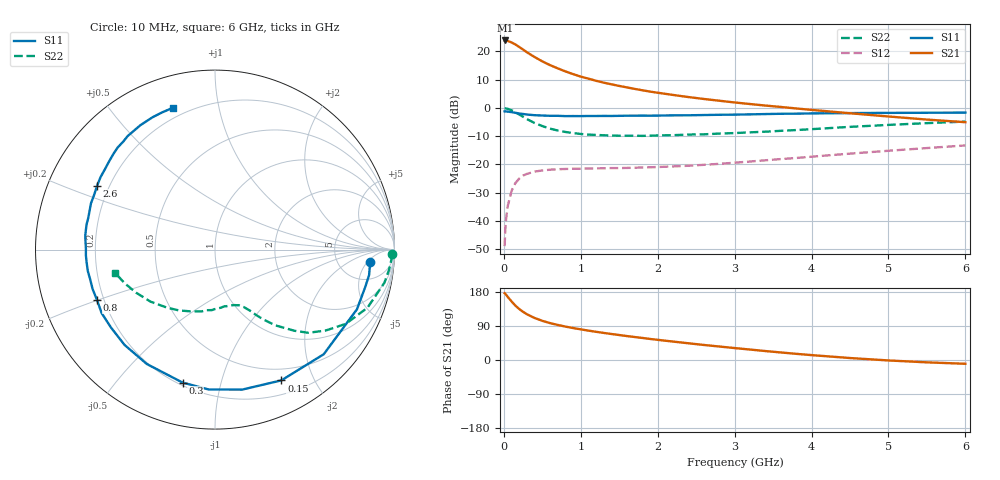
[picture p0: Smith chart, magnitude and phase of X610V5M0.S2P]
! SIEMENS Small Signal Semiconductors
! BFP193W
! Si NPN RF Bipolar Junction Transistor in SOT343
! VCE = 10 V  IC = 5 mA
! Common Emitter S-Parameters:  April 1994
# GHz  S  MA  R  50
!  f  S11  S21  S12  S22
! GHz  MAG  ANG  MAG  ANG  MAG  ANG  MAG  ANG
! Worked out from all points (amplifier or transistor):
!   40 points, 10 MHz to 6 GHz, reference 50 ohm
!   highest |S21| = 23.8 dB at 20 MHz (marker M1)
!   |S21| within 3 dB of that: start of sweep to 237.7 MHz
!   unconditionally stable (mu >= 1): 1.756 GHz to 4.541 GHz
!   at 200 MHz: K = 0.14, MSG = 23.2 dB, |S12| = -25.0 dB
!   at 1.5 GHz: K = 0.90, MSG = 14.5 dB, |S12| = -21.3 dB
!   at 6 GHz: K = 0.92, MSG = 4.1 dB, |S12| = -13.3 dB
!   S11 on the Smith chart (normalised r, x): 10 MHz: 11, -6; 150 MHz: 0.36, -1.57; 300 MHz: 0.22, -0.76; 800 MHz: 0.17, -0.20; 2.6 GHz: 0.15, +0.25; 6 GHz: 0.15, +0.74
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0.01  0.8672 -4.5  15.48 176.3  0.0036 85.0  0.9883 -1.5
0.02  0.8702 -9.3  15.52 174.5  0.0074 83.6  0.9813 -4.7
0.05  0.858 -22.8  15.22 166.8  0.0182 77.0  0.9617 -11.1
0.1  0.8408 -43.9  14.33 154.6  0.034 66.7  0.9089 -20.9
0.15  0.8171 -63.1  13.19 143.5  0.0469 57.8  0.8376 -29.6
0.2  0.7946 -79.0  11.89 134.5  0.0563 50.8  0.7635 -36.2
0.25  0.78 -92.6  10.71 127.1  0.0636 44.8  0.6967 -41.7
0.3  0.7626 -103.7  9.602 120.7  0.0682 39.9  0.633 -45.6
0.4  0.742 -120.8  7.902 110.9  0.0748 33.2  0.5403 -51.4
0.5  0.7322 -133.5  6.64 103.4  0.0784 29.0  0.4767 -55.1
0.6  0.7241 -143.2  5.692 97.4  0.0808 26.1  0.4301 -57.9
0.8  0.715 -156.8  4.405 88.2  0.0832 23.2  0.3753 -61.7
1  0.7149 -166.5  3.567 80.9  0.0842 21.7  0.346 -65.4
1.1  0.7187 -170.5  3.28 77.5  0.0848 21.6  0.3366 -66.9
1.3  0.72 -177.5  2.789 71.4  0.0855 21.9  0.3276 -70.6
1.6  0.727 173.8  2.298 63.1  0.0869 24.0  0.3214 -76.1
2.2  0.7375 159.6  1.691 48.6  0.0924 29.2  0.3291 -88.9
2.6  0.747 151.6  1.437 39.7  0.0985 33.1  0.3407 -97.8
3.2  0.7675 140.4  1.169 27.6  0.1126 37.6  0.3692 -111.1
4.5  0.8083 120.9  0.803 5.2  0.1554 40.4  0.4617 -141.1
5.5  0.8194 111.0  0.621 -6.2  0.1949 37.8  0.5374 -159.6
6  0.8246 106.3  0.558 -10.0  0.2167 36.0  0.5723 -167.1
